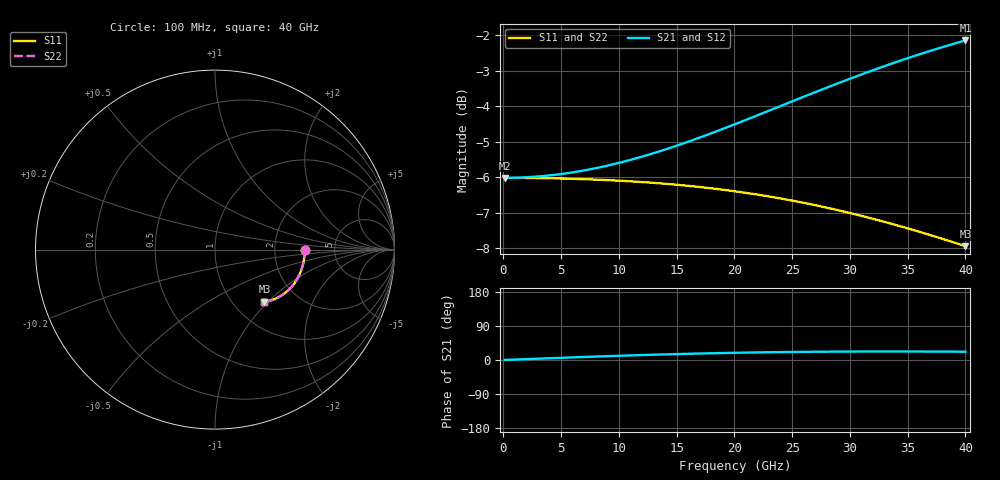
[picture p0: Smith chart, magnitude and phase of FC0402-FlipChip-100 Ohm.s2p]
!Vishay Thin-Film
!FC Family
!Case Size 0402
!Assembly Style Flip-Chip
!10/21/2015
!thinfilm@vishay.com
# GHz S MA R 50
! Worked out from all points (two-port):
!   101 points, 100 MHz to 40 GHz, reference 50 ohm
!   highest |S21| = -2.15 dB at 40 GHz (marker M1); lowest = -6.0 dB at 100 MHz (marker M2)
!   |S21| within 3 dB of the highest: 14.66 GHz to end of sweep
!   lowest |S11| = -7.9 dB at 40 GHz (marker M3), VSWR 2.34, Z = 68.9 - j47.7 ohm
!   |S11| at or under -10 dB: nowhere
!   |S22| runs from -7.9 to -6.0 dB; largest |S21 - S12| = 0
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0.1  0.5 -0.1  0.5 0.1  0.5 0.1  0.5 -0.1
1.696  0.4999 -2.0  0.5007 2.0  0.5007 2.0  0.4999 -2.0
3.292  0.4995 -3.9  0.5027 3.8  0.5027 3.8  0.4995 -3.9
4.888  0.499 -5.7  0.506 5.6  0.506 5.6  0.499 -5.7
6.883  0.4979 -8.1  0.5118 7.9  0.5118 7.9  0.4979 -8.1
8.479  0.4968 -10.0  0.5179 9.6  0.5179 9.6  0.4968 -10.0
10.075  0.4954 -11.9  0.5252 11.2  0.5252 11.2  0.4954 -11.9
12.07  0.4931 -14.3  0.536 13.1  0.536 13.1  0.4931 -14.3
13.666  0.491 -16.2  0.5459 14.5  0.5459 14.5  0.491 -16.2
16.858  0.4856 -20.0  0.5687 17.0  0.5687 17.0  0.4856 -20.0
20.05  0.4786 -23.9  0.595 19.0  0.595 19.0  0.4786 -23.9
22.045  0.4734 -26.3  0.6129 20.0  0.6129 20.0  0.4734 -26.3
23.641  0.4688 -28.3  0.6278 20.7  0.6278 20.7  0.4688 -28.3
25.237  0.4637 -30.2  0.643 21.3  0.643 21.3  0.4637 -30.2
26.833  0.4582 -32.1  0.6585 21.7  0.6585 21.7  0.4582 -32.1
28.828  0.4507 -34.4  0.678 22.1  0.678 22.1  0.4507 -34.4
30.424  0.4444 -36.3  0.6935 22.3  0.6935 22.3  0.4444 -36.3
32.02  0.4377 -38.1  0.7089 22.4  0.7089 22.4  0.4377 -38.1
33.616  0.4307 -39.9  0.7241 22.4  0.7241 22.4  0.4307 -39.9
35.212  0.4235 -41.6  0.7389 22.4  0.7389 22.4  0.4235 -41.6
36.808  0.4161 -43.3  0.7533 22.3  0.7533 22.3  0.4161 -43.3
40  0.4007 -46.5  0.7806 21.9  0.7806 21.9  0.4007 -46.5
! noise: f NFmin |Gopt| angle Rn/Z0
0.1  2.893e-15  1  -8.538e-07  2
4.489  9.643e-16  1  2.406e-15  1.944
8.878  0  1  -4.933e-15  1.791
13.27  1.436e-07  1  -2.575e-15  1.569
17.66  -2.411e-15  1  -8.538e-07  1.316
22.05  9.752e-08  1  2.185e-14  1.066
26.43  7.696e-08  1  1.324e-14  0.8409
30.82  9.643e-16  1  1.502e-14  0.6531
35.21  9.643e-16  1  2.895e-15  0.5031
40  9.643e-16  1  -1.708e-06  0.3778
